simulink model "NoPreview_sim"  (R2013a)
settings: Solver=ode45  StartTime=0.0  StopTime=60  RelTol=1e-3
undefined symbols (not defined in the file or in its folder): A, B, Bw, C_all, x0

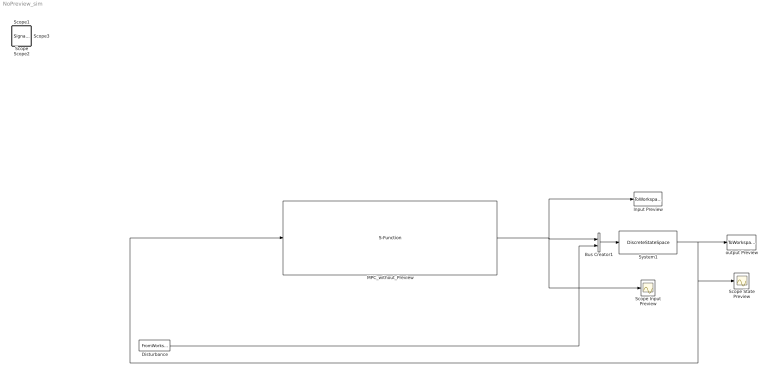
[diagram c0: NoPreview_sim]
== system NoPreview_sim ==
  Bus Creator1 : BusCreator  Inputs=2
  Disturbance : FromWorkspace  VariableName=[time, Road]  SampleTime=0
  Input Preview : ToWorkspace  VariableName=input_u_nopre  SampleTime=-1  SaveFormat=Timeseries
  MPC_without_Preview : S-Function  FunctionName=MPC_without_Preview_simulinkBlock  EnableBusSupport=off
  Scope Input Preview : Scope
  Scope State Preview : Scope
  System1 : DiscreteStateSpace  A=A  B=[B, Bw]  C=C_all  D=zeros(2,2)  X0=x0
  output Preview : ToWorkspace  VariableName=state_x_nopre  SampleTime=-1  SaveFormat=Timeseries
  Scope : SignalViewerScope  IOType=viewer  ZoomMode=yonly  RefreshTime=0.035000
  Scope1 : SignalViewerScope  IOType=viewer  RefreshTime=0.035000
  Scope2 : SignalViewerScope  IOType=viewer  RefreshTime=0.035000
  Scope3 : SignalViewerScope  IOType=viewer  RefreshTime=0.035000
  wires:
  MPC_without_Preview/1 -> Input Preview/1, Scope Input Preview/1, Bus Creator1/1
  System1/1 -> MPC_without_Preview/1, Scope State Preview/1, output Preview/1
  Bus Creator1/1 -> System1/1
  Disturbance/1 -> Bus Creator1/2
